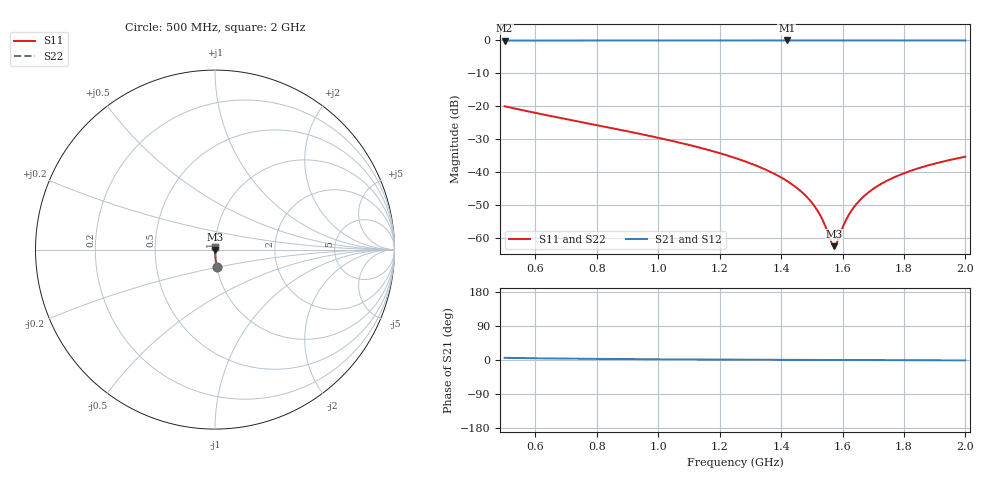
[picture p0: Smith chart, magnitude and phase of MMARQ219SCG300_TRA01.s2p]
! MMARQ219SCG300_TRA01  S-PARAMETER MODEL  ( General Type )
! Model Generated by TAIYO YUDEN Corporation (http://www.ty-top.com)
! Version 1.0
! TAIYO YUDEN Control No. 150609
! Copyright(c) 2015 TAIYO YUDEN CO.,LTD. All Rights Reserved.
! Product Description (link to TY-COMPAS)
! https://ds.yuden.co.jp/TYCOMPAS/or/detail?pn=MMARQ219SCG300JTRA01&u=M
! Products Name : Multilayer Ceramic Capacitors
! Characteristics :
!  Capacitance : 30 pF , Rated Voltage : 250V , TCC : CG / C0G
!  Case Size : 2.0 x 1.25 / 0.079 x 0.049 [mm/inch] , Thickness : 0.85 / 0.033 [mm/inch]
!  (Conditions: Temperature = 25 degC , DC Bias Current/Voltage = 0A / 0V)
! External Node Assignments :
!  1  o---| |---o  2
! GND o---------o GND
! Frequency Range : 500MHz  -  2GHz  [ 401 STEP ]
# MHz S RI R 50
! Freq[MHz].  S11 Real  S11 Imag  S21 Real  S21 Imag  S12 Real  S12 Imag  S22 Real  S22 Imag
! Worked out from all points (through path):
!   401 points, 500 MHz to 2 GHz, reference 50 ohm
!   highest |S21| = -0.01 dB at 1.419 GHz (marker M1); lowest = 0.0 dB at 500 MHz (marker M2)
!   group delay of S21, straight-line fit = 10.9 ps
!   lowest |S11| = -62.6 dB at 1.573 GHz (marker M3), VSWR 1.00, Z = 50.1 - j0.00193 ohm
!   |S11| at or under -10 dB: start of sweep to end of sweep
!   |S22| runs from -62.6 to -20.0 dB; largest |S21 - S12| = 0
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500  0.0103 -0.0993  0.9897 0.0993  0.9897 0.0993  0.0103 -0.0993
751.25  0.00367 -0.057  0.9963 0.057  0.9963 0.057  0.00367 -0.057
1002.5  0.0016 -0.0329  0.9984 0.0329  0.9984 0.0329  0.0016 -0.0329
1141.25  0.00111 -0.023  0.9989 0.023  0.9989 0.023  0.00111 -0.023
1250  0.000894 -0.0163  0.9991 0.0163  0.9991 0.0163  0.000894 -0.0163
1343.75  0.000787 -0.0111  0.9992 0.0111  0.9992 0.0111  0.000787 -0.0111
1418.75  0.000744 -0.00728  0.9993 0.00728  0.9993 0.00728  0.000744 -0.00728
1463.75  0.000733 -0.00507  0.9993 0.00507  0.9993 0.00507  0.000733 -0.00507
1501.25  0.000731 -0.00329  0.9993 0.00329  0.9993 0.00329  0.000731 -0.00329
1527.5  0.000734 -0.00206  0.9993 0.00206  0.9993 0.00206  0.000734 -0.00206
1542.5  0.000736 -0.00138  0.9993 0.00138  0.9993 0.00138  0.000736 -0.00138
1561.25  0.000741 -0.000525  0.9993 0.000525  0.9993 0.000525  0.000741 -0.000525
1572.5  0.000744 -1.93e-05  0.9993 1.93e-05  0.9993 1.93e-05  0.000744 -1.93e-05
1576.25  0.000746 0.000148  0.9993 -0.000148  0.9993 -0.000148  0.000746 0.000148
1583.75  0.000748 0.000483  0.9993 -0.000483  0.9993 -0.000483  0.000748 0.000483
1602.5  0.000756 0.00131  0.9992 -0.00131  0.9992 -0.00131  0.000756 0.00131
1617.5  0.000763 0.00197  0.9992 -0.00197  0.9992 -0.00197  0.000763 0.00197
1647.5  0.000779 0.00326  0.9992 -0.00326  0.9992 -0.00326  0.000779 0.00326
1692.5  0.000809 0.00516  0.9992 -0.00516  0.9992 -0.00516  0.000809 0.00516
1752.5  0.000859 0.00762  0.9991 -0.00762  0.9991 -0.00762  0.000859 0.00762
1861.25  0.000973 0.0119  0.999 -0.0119  0.999 -0.0119  0.000973 0.0119
2000  0.00116 0.017  0.9988 -0.017  0.9988 -0.017  0.00116 0.017
